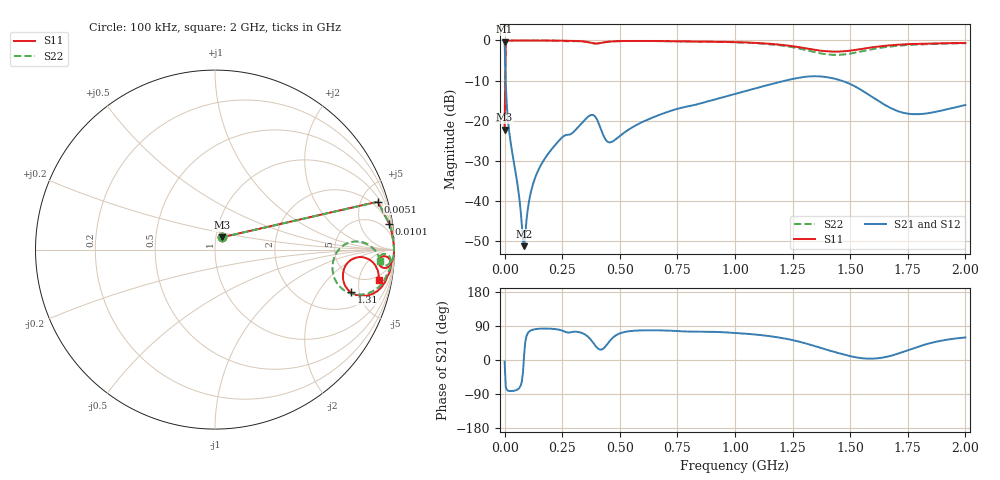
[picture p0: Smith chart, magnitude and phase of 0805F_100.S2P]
! Network Analyzer HP8753ES.07.68: Mar 08, 2001 Serial No. US39171556
! 21 Feb 2006  13:47:39
! Frequency  S11  S21  S12  S22
# HZ  S  RI R  50
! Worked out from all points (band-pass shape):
!   401 points, 100 kHz to 2 GHz, reference 50 ohm
!   highest |S21| = -0.30 dB at 100 kHz (marker M1); lowest = -51.2 dB at 85.1 MHz (marker M2)
!   |S21| within 3 dB of the highest: start of sweep to 1.508 MHz
!   lowest |S11| = -22.2 dB at 100 kHz (marker M3), VSWR 1.17, Z = 53.4 + j7.32 ohm
!   |S11| at or under -10 dB: start of sweep to 2.908 MHz
!   |S22| runs from -22.2 to 0.0 dB; largest |S21 - S12| = 0.00094
!   S11 on the Smith chart (normalised r, x): 100 kHz: 1.07, +0.15; 5.1 MHz: 1.32, +6.68; 10.1 MHz: 2, +13; 1.31 GHz: 3.20, -4.12; 2 GHz: 4, -9
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100000  0.0374 0.0682  0.9634 -0.0663  0.9638 -0.0671  0.0373 0.0682
5099750  0.9072 0.267  0.0927 -0.2678  0.0924 -0.2674  0.9075 0.2664
1.00995e7  0.971 0.145  0.0289 -0.1455  0.0288 -0.1454  0.9712 0.1454
1.509925e7  0.9847 0.0974  0.0153 -0.0977  0.0153 -0.0976  0.9845 0.0974
2.509875e7  0.9919 0.0561  0.00786 -0.0563  0.00795 -0.0562  0.992 0.0563
6.0097e7  0.9966 0.0127  0.0032 -0.0129  0.00323 -0.0129  0.9969 0.0133
7.509625e7  0.9975 0.00366  0.00277 -0.00413  0.00278 -0.00408  0.9973 0.00485
8.509575e7  0.9974 -0.00143  0.00265 0.000747  0.00265 0.000797  0.9977 0.000244
1.150942e8  0.9973 -0.0136  0.00269 0.013  0.00268 0.0131  0.9972 -0.0114
1.550922e8  0.9966 -0.0281  0.00347 0.0271  0.00346 0.027  0.9966 -0.0253
2.40088e8  0.9907 -0.0577  0.0107 0.0573  0.0106 0.0573  0.9875 -0.0564
3.350832e8  0.9702 -0.0932  0.0298 0.0886  0.0297 0.0886  0.9695 -0.0791
3.850808e8  0.9164 -0.0868  0.0829 0.0834  0.083 0.0834  0.9178 -0.0743
4.60077e8  0.967 -0.0464  0.0327 0.043  0.0326 0.0431  0.9671 -0.0333
6.700665e8  0.9746 -0.1198  0.024 0.1156  0.0238 0.1155  0.9752 -0.104
1.00005e9  0.9289 -0.2071  0.0686 0.2052  0.0683 0.2052  0.9289 -0.1909
1.310034e9  0.7573 -0.238  0.2574 0.2422  0.2572 0.2423  0.7212 -0.2283
1.335033e9  0.7393 -0.2218  0.2787 0.2241  0.2783 0.2246  0.6968 -0.2076
1.485026e9  0.7325 -0.0816  0.2921 0.0644  0.2919 0.0649  0.6738 -0.023
1.670016e9  0.8646 -0.0589  0.1446 0.0258  0.1444 0.0263  0.8363 0.0365
1.79001e9  0.9 -0.1022  0.0999 0.0677  0.0996 0.0681  0.8897 -0.00281
2e9  0.9119 -0.1687  0.0798 0.1352  0.0792 0.1356  0.919 -0.0657
